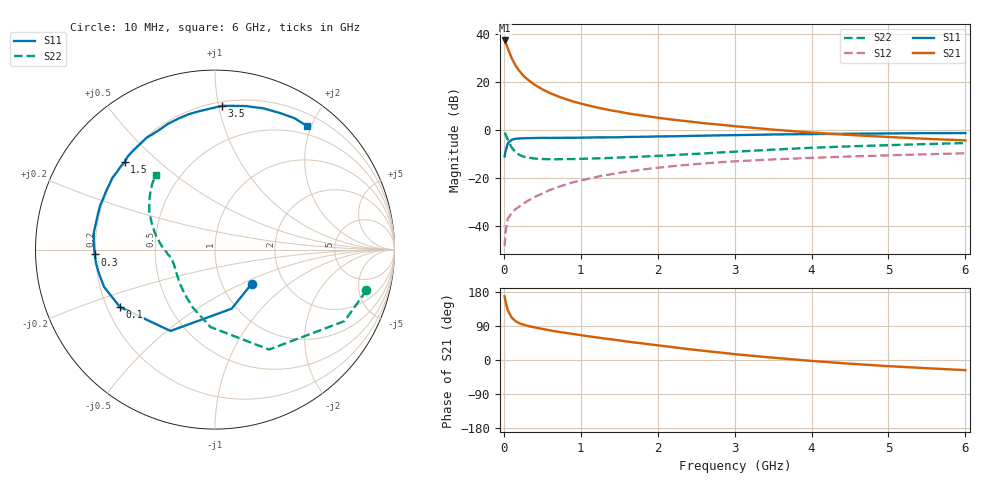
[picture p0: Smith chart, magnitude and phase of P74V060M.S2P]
! SIEMENS Small Signal Semiconductors
! BFP196
! Si NPN RF Bipolar Junction Transistor in SOT143
! VCE = 4 V  IC = 60 mA
! Common Emitter S-Parameters:  May  1996
# GHz  S  MA  R  50
!  f  S11  S21  S12  S22
! GHz  MAG  ANG  MAG  ANG  MAG  ANG  MAG  ANG
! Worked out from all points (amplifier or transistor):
!   36 points, 10 MHz to 6 GHz, reference 50 ohm
!   highest |S21| = 37.4 dB at 10 MHz (marker M1)
!   |S21| within 3 dB of that: start of sweep to 48.42 MHz
!   unconditionally stable (mu >= 1): 428.6 MHz to 4.342 GHz
!   at 250 MHz: K = 0.86, MSG = 26.9 dB, |S12| = -30.9 dB
!   at 1.4 GHz: K = 1.09, MAG = 11.5 dB, |S12| = -18.5 dB
!   at 6 GHz: K = 0.97, MSG = 2.7 dB, |S12| = -9.8 dB
!   S11 on the Smith chart (normalised r, x): 10 MHz: 1.38, -0.57; 100 MHz: 0.25, -0.26; 300 MHz: 0.20, -0.02; 1.5 GHz: 0.20, +0.39; 3.5 GHz: 0.23, +1.03; 6 GHz: 0.37, +1.93
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0.01  0.2791 -42.6  74.25 167.8  0.0037 78.9  0.8738 -15.1
0.02  0.342 -74.2  68.94 155.9  0.0069 71.9  0.8243 -28.9
0.05  0.5168 -118.7  51.78 131.9  0.0138 54.3  0.6331 -61.6
0.1  0.6186 -148.8  32.13 112.5  0.0181 50.0  0.4322 -93.3
0.15  0.6521 -161.4  22.54 103.0  0.0219 51.0  0.3444 -111.4
0.2  0.6604 -168.6  17.27 97.3  0.0248 54.0  0.3017 -123.5
0.25  0.6676 -173.8  13.86 93.4  0.0285 56.2  0.2786 -132.8
0.3  0.6709 -177.7  11.64 90.5  0.0321 58.8  0.2662 -138.9
0.4  0.6775 176.3  8.801 86.0  0.0395 61.8  0.252 -148.2
0.5  0.6815 171.5  7.049 82.1  0.0467 62.7  0.2458 -154.0
0.6  0.6797 166.7  5.885 78.2  0.0555 63.4  0.2438 -158.1
0.7  0.6819 162.8  5.057 74.6  0.0634 63.4  0.2436 -161.3
0.8  0.6856 159.1  4.427 71.6  0.0716 62.7  0.245 -163.9
0.9  0.6849 155.6  3.938 68.6  0.0798 62.4  0.2455 -166.1
1.1  0.6913 148.4  3.236 62.6  0.0953 60.7  0.2509 -169.2
1.5  0.7013 135.9  2.399 51.7  0.1263 55.7  0.264 -174.3
2.2  0.7334 116.0  1.633 33.8  0.1746 45.4  0.2971 176.1
2.8  0.7683 101.0  1.288 20.0  0.2097 36.4  0.3371 166.8
3.5  0.8025 87.1  1.013 6.0  0.2414 26.5  0.3865 156.5
4.5  0.8322 71.0  0.783 -9.8  0.2781 14.5  0.4528 144.0
5.5  0.8559 58.7  0.65 -21.7  0.3095 3.7  0.5066 133.6
6  0.8581 53.4  0.604 -26.8  0.3246 -2.0  0.5312 128.6
